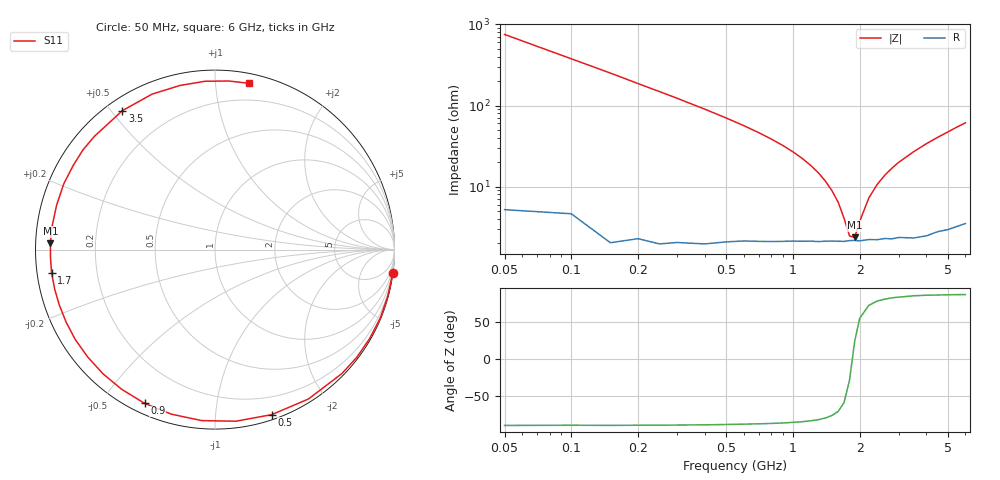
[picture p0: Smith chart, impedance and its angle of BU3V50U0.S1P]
! Infineon Technologies  Discrete & RF Semiconductors
! BB 833
! Si Tuning Diode in SOD323
! VR = 3.5 V
! S-Parameters:  June  1999
# GHz  S  MA  R  50
!  f  S11
! GHz  MAG  ANG
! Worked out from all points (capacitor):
!   34 points, 50 MHz to 6 GHz, reference 50 ohm
!   read as one part to ground: C = 4.21 pF near 50 MHz
!   lowest |Z| = 2.36 ohm at 1.9 GHz (marker M1)
!   series resonance near 1.855 GHz, so ESL is about 1.7 nH
!   S11 on the Smith chart (normalised r, x): 50 MHz: 0, -15; 500 MHz: 0.04, -1.40; 900 MHz: 0.04, -0.64; 1.7 GHz: 0.04, -0.07; 3.5 GHz: 0.05, +0.53; 6 GHz: 0.07, +1.22
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0.05  0.9991 -7.6
0.15  0.9969 -22.5
0.2  0.9939 -30.0
0.3  0.9885 -44.3
0.4  0.9818 -58.0
0.5  0.9724 -71.0
0.6  0.9632 -83.1
0.7  0.9556 -94.4
0.8  0.9486 -104.9
0.9  0.9421 -114.6
1  0.936 -123.7
1.1  0.9319 -132.1
1.2  0.9279 -139.9
1.3  0.9258 -147.2
1.4  0.9227 -154.0
1.6  0.9201 -166.2
1.7  0.9196 -172.0
1.9  0.9173 177.8
2.2  0.9166 164.3
2.4  0.9188 156.5
2.8  0.9218 142.9
3  0.9217 136.8
3.5  0.9304 123.7
4  0.9345 112.0
4.5  0.9351 102.0
5  0.9395 93.4
5.5  0.9426 85.3
6  0.9455 78.6
